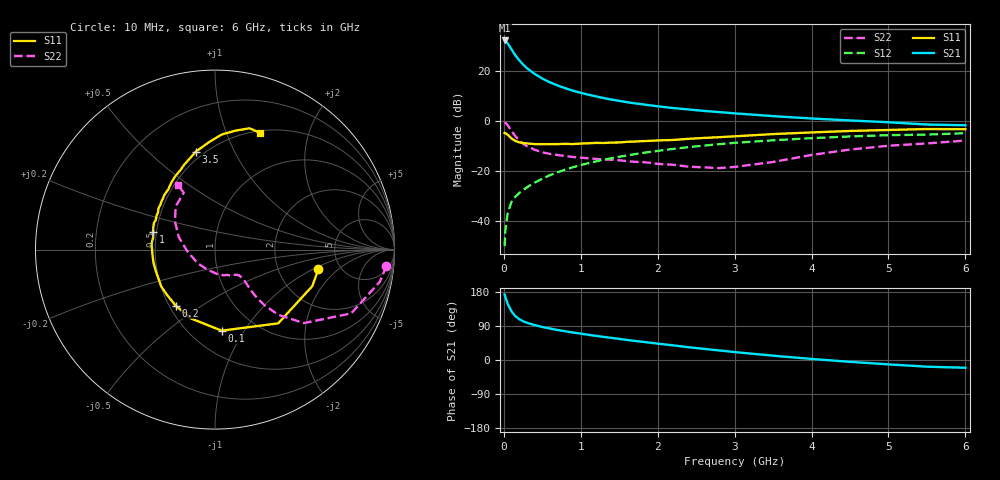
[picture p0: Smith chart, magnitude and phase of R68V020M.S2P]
! SIEMENS Small Signal Semiconductors
! BFR193
! Si NPN RF Bipolar Junction Transistor in SOT23
! VCE = 8 V  IC = 20 mA
! Common Emitter S-Parameters:  May  1996
# GHz  S  MA  R  50
!  f  S11  S21  S12  S22
! GHz  MAG  ANG  MAG  ANG  MAG  ANG  MAG  ANG
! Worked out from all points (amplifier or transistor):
!   36 points, 10 MHz to 6 GHz, reference 50 ohm
!   highest |S21| = 32.3 dB at 10 MHz (marker M1)
!   |S21| within 3 dB of that: start of sweep to 87.99 MHz
!   unconditionally stable (mu >= 1): 596.4 MHz to 2.126 GHz
!   at 250 MHz: K = 0.81, MSG = 25.1 dB, |S12| = -27.5 dB
!   at 1.4 GHz: K = 1.03, MAG = 10.7 dB, |S12| = -14.7 dB
!   at 6 GHz: K = 0.94, MSG = 1.6 dB, |S12| = -4.7 dB
!   lowest NFmin = 1.40 dB at 450 MHz
!   S11 on the Smith chart (normalised r, x): 10 MHz: 3.42, -1.14; 100 MHz: 0.70, -0.80; 200 MHz: 0.54, -0.39; 1 GHz: 0.48, +0.11; 3.5 GHz: 0.45, +0.72; 6 GHz: 0.52, +1.32
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0.01  0.5862 -10.8  41.38 172.7  0.0032 84.8  0.9591 -5.5
0.02  0.5789 -20.6  40.41 165.9  0.0065 77.1  0.9359 -11.0
0.05  0.5412 -49.4  36.23 148.4  0.0148 71.3  0.8379 -25.1
0.1  0.4532 -85.3  27.39 128.2  0.0246 64.1  0.6424 -39.6
0.15  0.4061 -109.2  20.83 115.6  0.0312 61.2  0.5069 -45.8
0.2  0.3813 -125.1  16.67 107.9  0.0369 62.1  0.4177 -48.3
0.25  0.3672 -137.4  13.66 102.3  0.0423 63.6  0.3577 -49.0
0.3  0.3629 -145.6  11.58 98.2  0.048 65.2  0.3203 -48.8
0.4  0.3511 -159.2  8.893 92.2  0.0596 66.9  0.2709 -47.7
0.5  0.3503 -167.7  7.161 87.1  0.0714 67.7  0.2401 -46.6
0.6  0.3496 -174.6  6.023 83.0  0.084 68.2  0.2235 -46.2
0.7  0.3511 179.4  5.207 79.1  0.0962 68.2  0.2121 -46.4
0.8  0.3551 174.4  4.576 75.7  0.1086 67.7  0.2018 -46.8
1  0.3592 164.3  3.714 69.5  0.1338 66.7  0.188 -48.5
1.1  0.3647 160.7  3.405 66.5  0.1461 65.9  0.1829 -50.6
1.3  0.369 153.9  2.917 60.9  0.1715 63.8  0.1731 -54.3
1.6  0.3899 143.8  2.414 52.9  0.2082 60.4  0.1605 -62.5
2.2  0.4246 127.8  1.845 38.6  0.2809 52.9  0.1356 -85.9
3.5  0.5564 101.0  1.272 11.4  0.4183 33.8  0.1542 -176.4
4.5  0.6426 86.6  1.043 -4.8  0.4998 19.7  0.2729 144.8
5.5  0.7028 74.1  0.864 -17.6  0.5433 5.5  0.3619 118.7
6  0.697 68.9  0.835 -20.5  0.5793 1.4  0.4132 120.0
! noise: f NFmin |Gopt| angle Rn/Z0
0.45  1.4  0.3  160  0.1
0.9  1.45  0.34  172  0.11
1.8  2.2  0.56  -148  0.2
